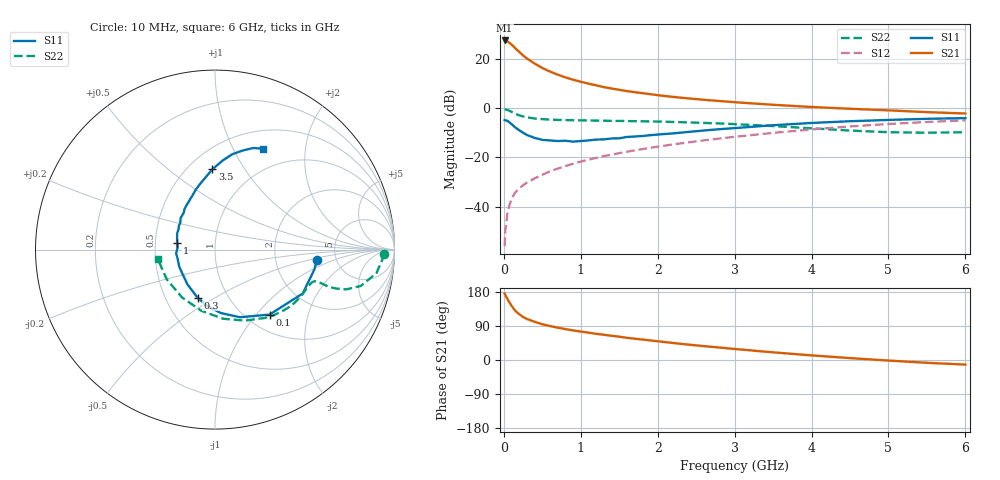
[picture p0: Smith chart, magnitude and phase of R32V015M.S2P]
! SIEMENS Small Signal Semiconductors
! BFR181
! Si NPN RF Bipolar Junction Transistor in SOT23
! VCE = 2 V  IC = 15 mA
! Common Emitter S-Parameters:  May  1996
# GHz  S  MA  R  50
!  f  S11  S21  S12  S22
! GHz  MAG  ANG  MAG  ANG  MAG  ANG  MAG  ANG
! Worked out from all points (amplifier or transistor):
!   36 points, 10 MHz to 6 GHz, reference 50 ohm
!   highest |S21| = 27.3 dB at 10 MHz (marker M1)
!   |S21| within 3 dB of that: start of sweep to 143.9 MHz
!   unconditionally stable (mu >= 1): 378.1 MHz to 3.016 GHz
!   at 250 MHz: K = 0.84, MSG = 26.3 dB, |S12| = -31.3 dB
!   at 1.4 GHz: K = 1.18, MAG = 10.8 dB, |S12| = -18.9 dB
!   at 6 GHz: K = 0.93, MSG = 1.4 dB, |S12| = -5.0 dB
!   S11 on the Smith chart (normalised r, x): 10 MHz: 3.54, -0.62; 100 MHz: 1.26, -1.18; 300 MHz: 0.72, -0.42; 1 GHz: 0.65, +0.05; 3.5 GHz: 0.65, +0.73; 6 GHz: 0.72, +1.32
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0.01  0.5709 -5.9  23.25 175.6  0.0016 97.3  0.942 -1.4
0.02  0.5647 -11.3  23.04 171.3  0.0034 82.2  0.9334 -3.5
0.05  0.5464 -26.6  22.11 159.7  0.0082 78.1  0.9088 -8.3
0.1  0.4726 -50.0  19.21 143.0  0.0146 70.9  0.8371 -14.0
0.15  0.4018 -69.7  16.11 129.6  0.0197 67.5  0.7628 -16.9
0.2  0.3553 -84.7  13.66 120.9  0.0236 66.7  0.7103 -17.8
0.25  0.316 -98.3  11.59 113.6  0.0273 66.5  0.6732 -18.1
0.3  0.2844 -110.0  10.04 108.3  0.0309 67.1  0.6461 -17.9
0.4  0.2478 -128.0  7.916 100.8  0.0377 68.6  0.6132 -17.5
0.5  0.2262 -143.1  6.445 94.4  0.0445 70.0  0.5949 -17.4
0.6  0.2206 -155.0  5.448 89.6  0.0524 71.2  0.5826 -17.6
0.7  0.2144 -166.1  4.723 85.3  0.0592 71.7  0.5743 -18.2
0.8  0.2175 -174.6  4.164 81.5  0.0666 71.9  0.5694 -18.8
1  0.2147 169.6  3.394 75.1  0.0823 72.7  0.5622 -20.7
1.1  0.2204 163.4  3.115 72.2  0.0899 72.9  0.5587 -21.7
1.3  0.2317 151.5  2.646 66.6  0.1062 72.5  0.5525 -24.2
1.6  0.2597 137.6  2.196 58.6  0.1305 71.4  0.5443 -28.3
2.2  0.3064 118.2  1.675 44.9  0.1834 68.2  0.5217 -38.0
3.5  0.448 91.8  1.161 20.2  0.3137 56.2  0.4302 -66.9
4.5  0.5396 79.8  0.964 5.0  0.4224 43.5  0.3493 -102.6
5.5  0.6046 69.4  0.824 -7.4  0.5209 28.7  0.3157 -148.3
6  0.6232 64.4  0.773 -12.1  0.5607 21.0  0.3235 -170.8
